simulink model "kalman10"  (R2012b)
settings: Solver=ode45  StartTime=0.0  StopTime=10.0  RelTol=1e-3
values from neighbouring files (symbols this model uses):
  A = [0 1 0 0 0 0    [beobachter_1.m]    (also in beobachter_2.m; beobachter_22.m; kalman_1.m = my_sys.a; kalman_10.m = my_sys.a)
  B = [0 1 0 0 0 0]'    [beobachter_1.m]    (also in beobachter_2.m; beobachter_22.m; kalman_1.m = my_sys.b; kalman_10.m = my_sys.b)
  C = [0 0 0 0 1 0]    [beobachter_1.m]    (also in beobachter_2.m; beobachter_22.m; kalman_1.m = my_sys.c; kalman_10.m = my_sys.c)
  dtn = 0.01    [kalman_1.m]    (also in kalman_10.m; kalman_11.m; kalman_12.m; kalman_d1.m)
  G = eye(2,2)    [kalman_1.m]    (also in kalman_10.m; kalman_11.m; kalman_12.m; kalman_d1.m = eye(3,3))
  Kest = kalman(P,1,0.01),    [LQG_1.m]    (also in ss_zwei_eing_1.m = kalman(sys2, Q, R))
  vnd = 1e-4    (= 0.0001)    [kalman_1.m]    (also in kalman_10.m; kalman_11.m; kalman_12.m; kalman_13.m = 0.01)
  vny = 1e-6    (= 1e-06)    [kalman_1.m]    (also in kalman_10.m; kalman_11.m = ', num2str(vny),' )']); kalman_12.m = ', num2str(vny),' )']); kalman_13.m = ', num2str(vny),' )']))
libraries: simulink x2

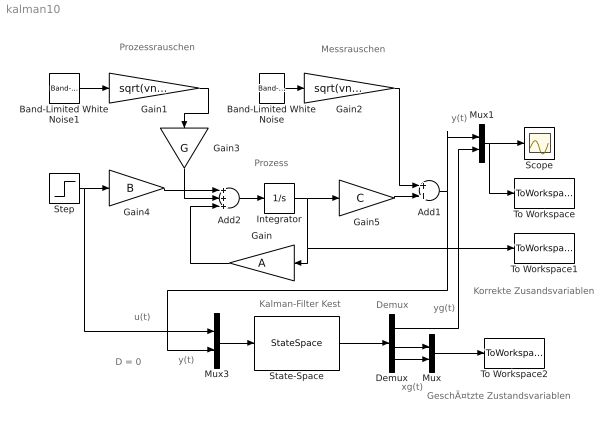
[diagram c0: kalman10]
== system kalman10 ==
  note: xg(t)
  note: y(t)
  note: u(t)
  note: Demux
  note: D = 0
  note: Kalman-Filter Kest
  note: Prozess
  note: Messrauschen
  note: Prozessrauschen
  note: yg(t)
  note: y(t)
  note: GeschÃ¤tzte Zustandsvariablen
  note: Korrekte Zusandsvariablen
  Add1 : Sum
  Add2 : Sum  Inputs=+++
  Band-Limited White Noise : simulink/Sources/Band-Limited White Noise  Cov=dtn  Ts=dtn  seed=[23341]
  Band-Limited White Noise1 : simulink/Sources/Band-Limited White Noise  Cov=[dtn, dtn]  Ts=dtn  seed=[296441, 37829]
  Demux : Demux  Outputs=3
  Gain : Gain  Gain=A  Multiplication=Matrix(K*u)
  Gain1 : Gain  Gain=sqrt(vnd/dtn)
  Gain2 : Gain  Gain=sqrt(vny/dtn)
  Gain3 : Gain  Gain=G  Multiplication=Matrix(K*u)
  Gain4 : Gain  Gain=B  Multiplication=Matrix(K*u)
  Gain5 : Gain  Gain=C  Multiplication=Matrix(K*u)
  Integrator : Integrator
  Mux : Mux  Inputs=2
  Mux1 : Mux  Inputs=2
  Mux3 : Mux  Inputs=2
  Scope : Scope
  State-Space : StateSpace  A=Kest.a  B=Kest.b  C=Kest.c  D=Kest.d
  Step : Step  SampleTime=0
  To Workspace : ToWorkspace  VariableName=y  SaveFormat=Structure With Time
  To Workspace1 : ToWorkspace  VariableName=y1  SaveFormat=Structure With Time
  To Workspace2 : ToWorkspace  VariableName=y2  SaveFormat=Structure With Time
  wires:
  Band-Limited White Noise/1 -> Gain2/1
  Gain2/1 -> Add1/1
  Add2/1 -> Integrator/1
  Band-Limited White Noise1/1 -> Gain1/1
  Gain1/1 -> Gain3/1
  Gain/1 -> Add2/3
  Gain3/1 -> Add2/2
  Gain4/1 -> Add2/1
  Gain5/1 -> Add1/2
  Integrator/1 -> To Workspace1/1, Gain/1, Gain5/1
  Mux1/1 -> Scope/1, To Workspace/1
  Demux/1 -> Mux1/2
  Demux/2 -> Mux/1
  Demux/3 -> Mux/2
  Mux/1 -> To Workspace2/1
  Step/1 -> Mux3/1, Gain4/1
  State-Space/1 -> Demux/1
  Add1/1 -> Mux3/2, Mux1/1
  Mux3/1 -> State-Space/1
